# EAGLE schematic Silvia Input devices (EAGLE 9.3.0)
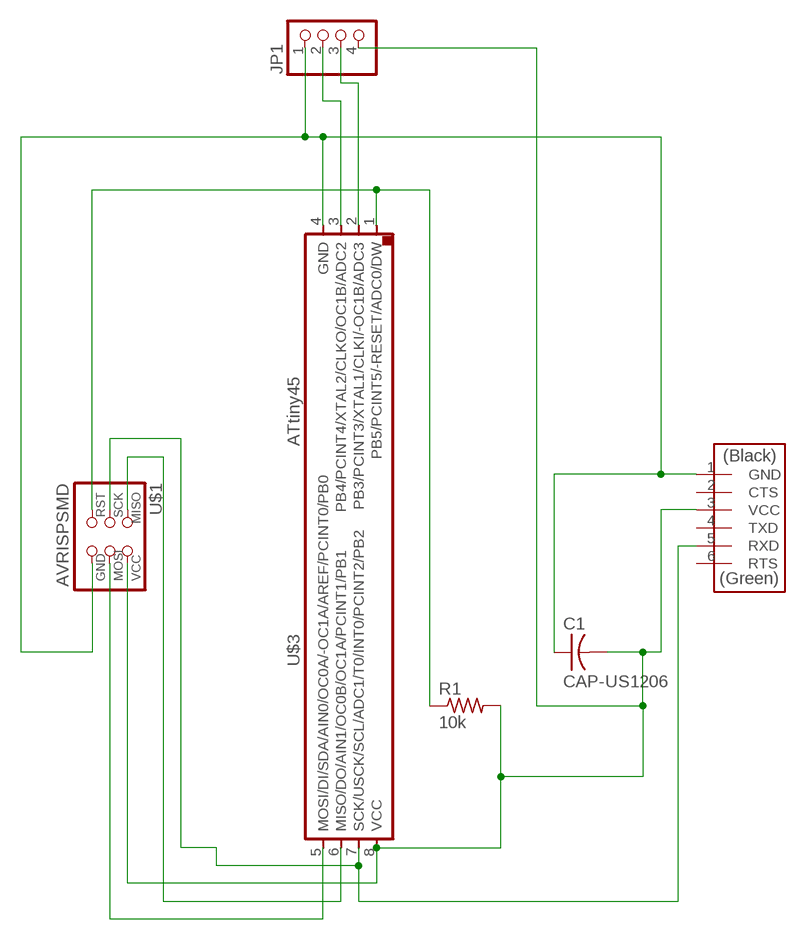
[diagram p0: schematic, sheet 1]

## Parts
C1  CAP-US1206  [C1206]
JP1  PINHD-1X4  [1X04]
R1  10k  RES-US1206FAB  [R1206FAB]
U$1  AVRISPSMD  [2X03SMD]
U$2  FTDI-SMD-HEADER  [1X06SMD]
U$3  ATTINY45SI  [SOIC8]

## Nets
N$1: C1.2 JP1.4 R1.2 U$1.2(VCC) U$2.3(VCC) U$3.8(VCC)
N$2: C1.1 JP1.1 U$1.6(GND) U$2.1(GND) U$3.4(GND)
N$4: U$1.3(SCK) U$2.5(RXD) U$3.7(SCK/USCK/SCL/ADC1/T0/INT0/PCINT2/PB2)
N$5: R1.1 U$1.5(RST) U$3.1(PB5/PCINT5/-RESET/ADC0/DW)
N$6: U$1.1(MISO) U$3.6(MISO/DO/AIN1/OC0B/OC1A/PCINT1/PB1)
N$7: U$1.4(MOSI) U$3.5(MOSI/DI/SDA/AIN0/OC0A/-OC1A/AREF/PCINT0/PB0)
N$9: JP1.2 U$3.3(PB4/PCINT4/XTAL2/CLKO/OC1B/ADC2)
N$10: JP1.3 U$3.2(PB3/PCINT3/XTAL1/CLKI/-OC1B/ADC3)
Unconnected: U$2.2(CTS) U$2.4(TXD) U$2.6(RTS)

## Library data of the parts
C1 = fab:CAP-US
JP1 = pinhead:PINHD-1X4: PIN HEADER
R1 = fab:RES-US: Resistor (US Symbol)
U$1 = fab:AVRISP
U$2 = fab:FTDI-SMD-HEADER
U$3 = fab:ATTINY45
